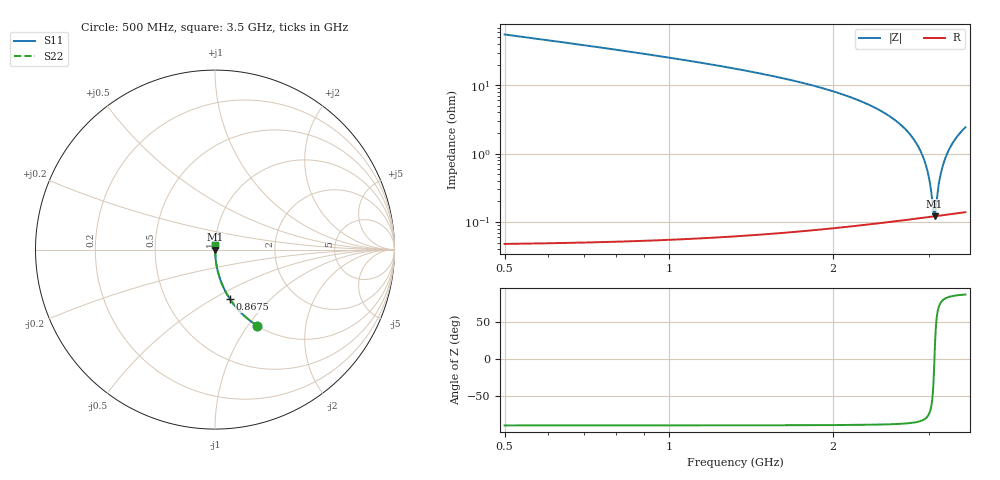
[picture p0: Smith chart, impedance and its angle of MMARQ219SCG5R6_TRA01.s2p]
! MMARQ219SCG5R6_TRA01  S-PARAMETER MODEL  ( General Type )
! Model Generated by TAIYO YUDEN Corporation (http://www.ty-top.com)
! Version 1.0
! TAIYO YUDEN Control No. 180601
! Copyright(c) 2018 TAIYO YUDEN CO.,LTD. All Rights Reserved.
! Product Description (link to TY-COMPAS)
! https://ds.yuden.co.jp/TYCOMPAS/or/detail?pn=MMARQ219SCG5R6CTRA01&u=M
! Products Name : Multilayer Ceramic Capacitors
! Characteristics :
!  Capacitance : 5.6 pF , Rated Voltage : 250V , TCC : CG / C0G
!  Case Size : 2.0 x 1.25 / 0.079 x 0.049 [mm/inch] , Thickness : 0.85 / 0.033 [mm/inch]
!  (Conditions: Temperature = 25 degC , DC Bias Current/Voltage = 0A / 0V)
! External Node Assignments :
!  1  o---| |---o  2
! GND o---------o GND
! Frequency Range : 500MHz  -  3500MHz  [ 401 STEP ]
# MHz S RI R 50
! Freq[MHz].  S11 Real  S11 Imag  S21 Real  S21 Imag  S12 Real  S12 Imag  S22 Real  S22 Imag
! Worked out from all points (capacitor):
!   401 points, 500 MHz to 3.5 GHz, reference 50 ohm
!   read as one part in series: C = 5.6 pF near 515 MHz
!   lowest |Z| = 121 mohm at 3.072 GHz (marker M1)
!   series resonance near 3.071 GHz, so ESL is about 480 pH
!   S11 on the Smith chart (normalised r, x): 500 MHz: 1.00, -1.11; 867.5 MHz: 1.00, -0.60; 3.5 GHz: 1.00, +0.05
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500  0.2347 -0.4234  0.7653 0.4234  0.7653 0.4234  0.2347 -0.4234
665  0.1427 -0.3491  0.8573 0.3491  0.8573 0.3491  0.1427 -0.3491
867.5  0.0837 -0.2761  0.9163 0.2761  0.9163 0.2761  0.0837 -0.2761
1002.5  0.0607 -0.2378  0.9393 0.2378  0.9393 0.2378  0.0607 -0.2378
1505  0.0208 -0.1404  0.9792 0.1404  0.9792 0.1404  0.0208 -0.1404
2000  0.00743 -0.0811  0.9926 0.0811  0.9926 0.0811  0.00743 -0.0811
2502.5  0.00243 -0.038  0.9976 0.038  0.9976 0.038  0.00243 -0.038
2690  0.00166 -0.0245  0.9983 0.0245  0.9983 0.0245  0.00166 -0.0245
2832.5  0.00133 -0.0149  0.9987 0.0149  0.9987 0.0149  0.00133 -0.0149
2937.5  0.00122 -0.0082  0.9988 0.0082  0.9988 0.0082  0.00122 -0.0082
2975  0.0012 -0.00586  0.9988 0.00586  0.9988 0.00586  0.0012 -0.00586
3005  0.0012 -0.00401  0.9988 0.00401  0.9988 0.00401  0.0012 -0.00401
3027.5  0.0012 -0.00264  0.9988 0.00264  0.9988 0.00264  0.0012 -0.00264
3057.5  0.0012 -0.000824  0.9988 0.000824  0.9988 0.000824  0.0012 -0.000824
3072.5  0.00121 7.72e-05  0.9988 -7.72e-05  0.9988 -7.72e-05  0.00121 7.72e-05
3087.5  0.00121 0.000974  0.9988 -0.000974  0.9988 -0.000974  0.00121 0.000974
3117.5  0.00123 0.00275  0.9988 -0.00275  0.9988 -0.00275  0.00123 0.00275
3140  0.00125 0.00408  0.9987 -0.00408  0.9987 -0.00408  0.00125 0.00408
3170  0.00128 0.00583  0.9987 -0.00583  0.9987 -0.00583  0.00128 0.00583
3215  0.00134 0.00843  0.9987 -0.00843  0.9987 -0.00843  0.00134 0.00843
3335  0.00155 0.0152  0.9985 -0.0152  0.9985 -0.0152  0.00155 0.0152
3500  0.00197 0.0241  0.998 -0.0241  0.998 -0.0241  0.00197 0.0241
